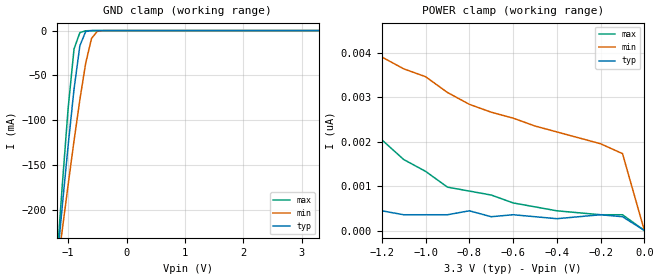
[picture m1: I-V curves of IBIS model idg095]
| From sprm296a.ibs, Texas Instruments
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[Model]   idg095
Model_type   Input
Polarity   Non-Inverting
| signals   A, Y
Vinl = 0.8V
Vinh = 2.0V
|   typ   min   max
C_comp   2.1548p   2.1455p   2.3140p
|   typ   min   max
[Temperature Range]   25   -40   125
|   typ   min   max
[Voltage Range]   3.30V   3.00V   3.60V
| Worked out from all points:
|   GND clamp passes 1 mA (typ) near -0.70 V on its own axis
[GND_clamp]
|   Voltage   I(typ)   I(min)   I(max)
-3.3V     -1.815A    -1.395A    -2.322A
-1.2V     -264.6mA   -272.7mA   -262.7mA
-1.1V     -194.9mA   -221.8mA   -171.5mA
-1V       -127.7mA   -171.7mA   -86.18mA
-900mV    -65.34mA   -123.1mA   -20.5mA
-800mV    -16.92mA   -77.05mA   -2.273mA
-700mV    -1.023mA   -36.39mA   -230.5uA
-600mV    -42.71uA   -8.724mA   -13.26uA
-500mV    -2.097uA   -764.8uA   -463.6nA
-300mV    -3.775nA   -2.577uA   -272pA
3.3V      222pA      2.087nA    310.9pA
[POWER_clamp]
|   Voltage   I(typ)   I(min)   I(max)
-3.3V     6.484nA    21.94nA    577.9nA
-3.1V     4.885nA    18.56nA    335.9nA
-2.8V     2.931nA    14.48nA    147.8nA
-2.4V     1.599nA    10.48nA    49.38nA
-1.6V     710.5pA    5.329nA    5.507nA
-1.5V     621.7pA    4.885nA    4.263nA
-1.4V     532.9pA    4.619nA    3.286nA
-1.2V     444.1pA    3.908nA    2.043nA
-900mV    355.3pA    3.109nA    977pA
-400mV    266.4pA    2.22nA     444.1pA
-100mV    310.9pA    1.732nA    355.3pA
0V        1pA        1pA        1pA
